ORGANIZATION_BLOCK MAIN:OB1
TITLE=Marcia/Arresto M.A.T.
//Simulatore: 00
//Versione: 1.0
//Data:26/02/2002
//
//-------------------- Descrizione Programma ---------------
// Gestione di un Marcia/Arresto completo di protezioni e segnalazioni
// risolto con istruzioni di assegnazione e autoritenuta software.
//
// Come prescritto dalle norme il relè termico FR dovrà
// intervenire direttamente in hardware alla diseccitazione del
// contattore KM; l'informazione dell'intervento viene portata al
// PLC mediante un ulteriore contatto del relè al fine di
// permettere al programma di disattivare le uscite e segnalarne
// l'intervento con la lampada gestita dall'uscita Q0.3.
// Il programma grazie all'interrogazione del contatto ausiliario
// di KM provvederà a resettare l'uscita anche quando per cause
// esterne (circuiti di sicurezza intervento termico)
// il contattore KM viene diseccitato.

BEGIN
NETWORK 1 //Comando Motore
//
LD Q0.0
A I0.2
O I0.1
A I0.0
A I0.3
= Q0.0

NETWORK 2 //Segnalazione Relè Termico
//
LDN I0.3
= Q0.3

NETWORK 3 //Segnalazione Marcia
//
LD Q0.0
= Q0.2

NETWORK 4 //Segnalazione Arresto
//
LDN Q0.0
= Q0.1

END_ORGANIZATION_BLOCK

